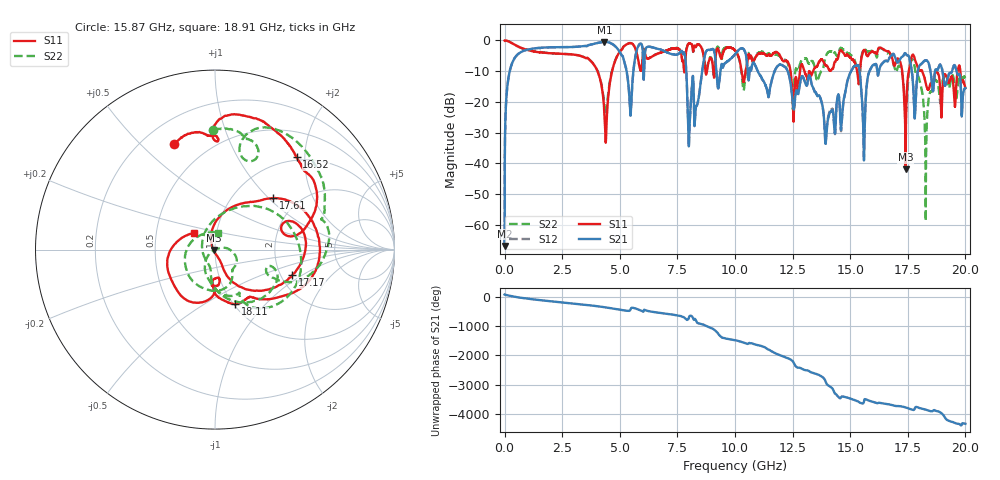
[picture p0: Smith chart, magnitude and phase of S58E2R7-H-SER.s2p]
!{S58E2R7}
!Johanson Technology Inc.
!www.johansontechnology.com
!Test Board Conditions:
!Substrate Type  RO4350B
!Substrate Thickness  60 mil
!Substrate Dk  3.66
!TL Type: GCPW
!TL Trace Width  115 mil
!TL Gap  52 mil
!Electrode orientation  Horizontal
!DUT TOPOLOGY	SERIES
!Mounting Pad LxW  55x428 mil
! Created Tue Apr 13 22:34:58 2021
# hz S ma R 50
! 2 Port Network Data from SP1.SP block
! freq  magS11  angS11  magS21  angS21  magS12  angS12  magS22  angS22
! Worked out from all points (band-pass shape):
!   20001 points, 300 kHz to 20 GHz, reference 50 ohm
!   highest |S21| = -0.46 dB at 4.329 GHz (marker M1); lowest = -66.9 dB at 300 kHz (marker M2)
!   |S21| within 3 dB of the highest: 794.2 MHz to 4.975 GHz (4.181 GHz wide, 145 % of centre); 6.1 GHz to 6.925 GHz (825.6 MHz wide, 12.7 % of centre)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
!   lowest |S11| = -41.9 dB at 17.41 GHz (marker M3), VSWR 1.02, Z = 49.2 - j0.261 ohm
!   |S11| at or under -10 dB: 4.032 GHz to 4.667 GHz (634.9 MHz wide, 14.6 % of centre); 18.13 GHz to 18.7 GHz (572.8 MHz wide, 3.11 % of centre); 18.75 GHz to 19.66 GHz (917.3 MHz wide, 4.78 % of centre)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
!   |S22| runs from -58.9 to 0.0 dB; largest |S21 - S12| = 0.017
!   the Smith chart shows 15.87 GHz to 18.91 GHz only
!   S11 on the Smith chart (normalised r, x): 15.87 GHz: 0.32, +0.64; 16.52 GHz: 0.94, +1.83; 17.17 GHz: 2.31, -0.82; 17.61 GHz: 1.51, +1.06; 18.11 GHz: 1.02, -0.69; 18.91 GHz: 0.78, +0.15
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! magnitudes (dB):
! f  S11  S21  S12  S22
! 300 kHz  0.0  -66.9  -67.0  -0.1
! 123.3 MHz  -0.2  -14.7  -14.6  -0.2
! 417.3 MHz  -1.3  -6.0  -5.9  -1.3
! 3.334 GHz  -5.1  -1.9  -1.9  -5.1
! 4.329 GHz  -23.3  -0.5  -0.5  -21.1
! 5.452 GHz  -0.9  -23.6  -23.5  -0.8
! 6.667 GHz  -4.2  -2.7  -2.7  -4.3
! 7.754 GHz  -7.0  -4.2  -4.2  -7.0
! 8.018 GHz  -0.9  -29.8  -29.8  -1.0
! 8.782 GHz  -10.1  -3.2  -3.2  -9.4
! 10 GHz  -3.2  -4.5  -4.5  -3.3
! 13.33 GHz  -11.1  -14.5  -14.4  -6.7
! 13.96 GHz  -8.2  -31.3  -31.0  -4.8
! 15.87 GHz  -4.0  -9.4  -9.5  -3.5
! 16.52 GHz  -3.3  -6.7  -6.6  -3.5
! 16.67 GHz  -3.5  -6.3  -6.1  -3.8
! 17.17 GHz  -6.9  -6.1  -6.0  -8.4
! 17.41 GHz  -41.9  -4.3  -4.3  -22.3
! 17.61 GHz  -7.3  -7.3  -7.2  -7.5
! 18.11 GHz  -9.8  -7.5  -7.5  -16.4
! 18.91 GHz  -16.6  -7.9  -7.9  -20.4
! 20 GHz  -15.5  -15.5  -15.5  -12.3
